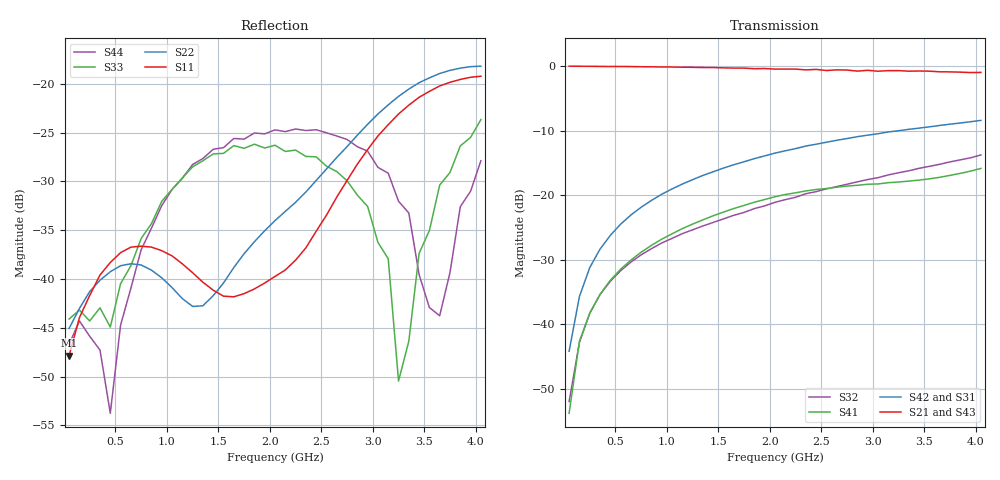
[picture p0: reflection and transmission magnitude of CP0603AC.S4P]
! Network Analyzer HP8720D.07.14 Serial No. US38111185
! 28 Apr 1999  02:06:29
! Frequency 	S11		S21		S31		S41		S12		S22		S23		S24		S13		S23		S33		S34		S14		S24		S34		S44
# HZ  S  DB R 50
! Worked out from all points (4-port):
!   41 points, 50 MHz to 4.05 GHz, reference 50 ohm
!   strongest paths, dB at 50 MHz, 1.05 GHz, 2.05 GHz, 3.05 GHz, 4.05 GHz:
!     S21: 0.0, -0.1, -0.4, -0.8, -1.0
!     S43: 0.0, -0.1, -0.5, -0.8, -1.0
!     S42: -44.2, -19.0, -13.5, -10.5, -8.4
!     S31: -43.4, -19.1, -13.5, -10.5, -8.3
!     S41: -53.8, -26.0, -20.2, -18.2, -15.8
!     S32: -52.0, -26.7, -21.1, -17.3, -13.7
!   lowest |S11| = -47.8 dB at 50 MHz (marker M1), VSWR 1.01, Z = 50.4 - j0.115 ohm
!   |S11| at or under -10 dB: start of sweep to end of sweep
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5e7  -47.85 -16.3  0.01 -1.2  -45.14 94.2  -55.13 93.7
     0.02 -0.9  -45.07 -3.2  -51.24 88.9  -45.72 94.4
     -43.41 89.2  -51.97 89.1  -44.10 2.1  -0.02 -1.1
     -53.79 86.3  -44.16 82.7  0.00 -0.9  -46.70 0.9
4.5e8  -38.31 -81.4  -0.04 -8.2  -26.24 81.3  -33.20 81.9
       -0.03 -8.4  -39.26 -67.3  -33.32 79.6  -26.19 81.0
       -26.23 81.2  -33.33 79.4  -44.93 69.6  -0.04 -8.2
       -33.17 81.9  -26.22 80.8  -0.04 -8.4  -53.77 81.3
9.5e8  -37.10 -107.8  -0.10 -17.5  -19.90 72.4  -26.81 73.4
       -0.11 -17.7  -39.88 -88.1  -27.40 70.5  -19.84 71.8
       -19.89 72.2  -27.39 70.4  -32.04 110.6  -0.12 -17.4
       -26.79 73.3  -19.83 71.6  -0.11 -17.6  -32.47 126.3
2.05e9  -39.74 -49.5  -0.40 -37.2  -13.54 53.6  -20.30 53.4
        -0.44 -37.5  -34.02 -20.4  -21.20 57.9  -13.53 52.4
        -13.50 53.3  -21.08 58.3  -26.29 118.7  -0.42 -37.0
        -20.22 53.6  -13.46 51.9  -0.47 -37.3  -24.72 131.0
3.25e9  -23.09 -0.7  -1.01 -59.0  -10.19 32.2  -18.00 34.9
        -0.67 -57.9  -21.29 -8.2  -16.63 40.0  -10.23 30.5
        -9.97 32.4  -16.50 39.9  -50.46 176.1  -1.03 -58.4
        -17.94 34.6  -9.99 30.1  -0.75 -57.4  -32.03 132.6
3.65e9  -20.21 -5.7  -1.35 -67.1  -9.43 25.4  -17.22 33.4
        -0.85 -64.9  -18.94 -13.4  -15.27 32.6  -9.51 23.6
        -9.15 26.5  -15.19 33.4  -30.37 -71.3  -1.34 -66.5
        -17.21 33.4  -9.17 23.8  -0.92 -64.4  -43.77 -87.6
4.05e9  -19.22 -7.6  -1.85 -75.1  -8.69 17.9  -15.86 30.5
        -0.95 -71.4  -18.19 -17.0  -13.97 22.9  -8.79 16.2
        -8.32 20.5  -13.74 25.2  -23.67 -81.0  -1.80 -74.6
        -15.83 31.6  -8.38 17.8  -1.03 -70.5  -27.88 -80.7
